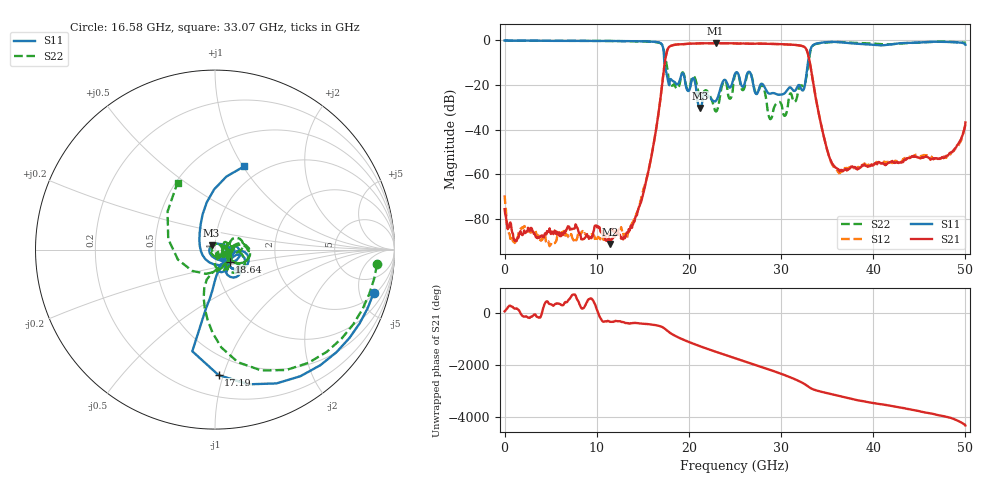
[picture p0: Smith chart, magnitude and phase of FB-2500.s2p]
! MARKI MICROWAVE INC.
! Email:  info@markimicrowave.com  Phone:  408-778-4200
! Model Number:  FB-2500  Date:  07/13
! Filename:		FB-2500.S2P  Version: 1.0
! Description:  2-port S-parameter data for Band Pass Filter FB-2500
! Frequency Measured: 	10 MHz to 50 GHz
! Measurements:		S11, S21, S12, S22
# Hz S  dB  R 50
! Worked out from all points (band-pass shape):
!   729 points, 10 MHz to 50 GHz, reference 50 ohm
!   highest |S21| = -1.25 dB at 22.9 GHz (marker M1); lowest = -91.1 dB at 11.49 GHz (marker M2)
!   |S21| within 3 dB of the highest: 17.67 GHz to 32.77 GHz (15.1 GHz wide, 59.9 % of centre)
!   lowest |S11| = -30.3 dB at 21.25 GHz (marker M3), VSWR 1.06, Z = 48.1 + j2.31 ohm
!   |S11| at or under -10 dB: 17.35 GHz to 32.92 GHz (15.56 GHz wide, 61.9 % of centre)
!   |S22| runs from -35.2 to 0.0 dB; largest |S21 - S12| = 0.0027
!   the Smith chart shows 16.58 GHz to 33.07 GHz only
!   S11 on the Smith chart (normalised r, x): 16.58 GHz: 2.21, -6.68; 17.19 GHz: 0.35, -0.96; 18.64 GHz: 1.16, -0.16; 33.07 GHz: 0.83, +1.01
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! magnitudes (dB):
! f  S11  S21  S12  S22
! 10 MHz  0.0  -75.5  -69.3  0.0
! 422.4 MHz  -0.1  -83.5  -85.8  -0.1
! 8.396 GHz  -0.2  -89.0  -85.7  -0.2
! 11.49 GHz  -0.3  -91.1  -86.7  -0.3
! 14.24 GHz  -0.4  -78.7  -78.6  -0.4
! 16.58 GHz  -0.8  -36.3  -36.3  -0.8
! 16.71 GHz  -0.9  -32.4  -32.4  -1.0
! 17.19 GHz  -3.1  -16.3  -16.3  -2.8
! 17.68 GHz  -16.8  -4.2  -4.2  -13.0
! 18.64 GHz  -19.5  -1.8  -1.8  -21.4
! 20.49 GHz  -17.0  -1.4  -1.4  -15.9
! 21.25 GHz  -30.3  -1.3  -1.3  -25.1
! 22.9 GHz  -27.2  -1.3  -1.2  -31.7
! 25.03 GHz  -14.8  -1.4  -1.4  -15.3
! 30.39 GHz  -23.7  -1.7  -1.7  -33.8
! 32.39 GHz  -22.4  -2.6  -2.6  -20.5
! 33.07 GHz  -6.2  -8.8  -8.8  -7.4
! 33.35 GHz  -2.7  -15.4  -15.4  -3.0
! 35.82 GHz  -0.7  -56.7  -57.0  -0.7
! 41.73 GHz  -1.9  -54.7  -54.9  -1.7
! 48.06 GHz  -0.7  -51.6  -51.7  -0.6
! 50 GHz  -1.9  -36.7  -36.5  -1.1
